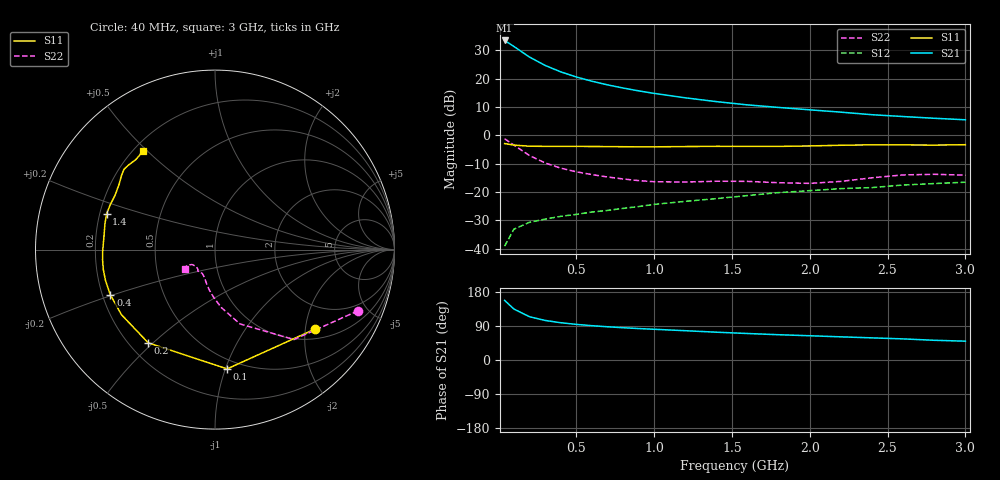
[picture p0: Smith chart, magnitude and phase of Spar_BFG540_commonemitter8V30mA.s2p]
! Filename:  BFG540J.S2P  Version:  3.0
! NXP part #: BFG540  Date: Feb 1992
! Bias condition: Vce=8V, Ic=30mA
! IN LINE PINNING: same data as with cross emitter pinning.
#  MHz  S  MA  R  50
! Freq  S11  S21  S12  S22  !GUM [dB]
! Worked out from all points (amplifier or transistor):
!   21 points, 40 MHz to 3 GHz, reference 50 ohm
!   highest |S21| = 33.4 dB at 40 MHz (marker M1)
!   |S21| within 3 dB of that: start of sweep to 123.3 MHz
!   unconditionally stable (mu >= 1): 825 MHz to end of sweep
!   at 300 MHz: K = 0.56, MSG = 27.1 dB, |S12| = -29.6 dB
!   at 1 GHz: K = 1.07, MAG = 18.0 dB, |S12| = -24.4 dB
!   at 3 GHz: K = 1.17, MAG = 8.5 dB, |S12| = -16.6 dB
!   lowest NFmin = 1.70 dB at 900 MHz
!   S11 on the Smith chart (normalised r, x): 40 MHz: 1.25, -2.25; 100 MHz: 0.42, -1.01; 200 MHz: 0.27, -0.48; 400 MHz: 0.23, -0.20; 1.4 GHz: 0.23, +0.15; 3 GHz: 0.24, +0.48
40  0.711 -38.6  46.95 157.3  0.011 71.0  0.866 -23.2
100  0.668 -84.2  36.73 134.4  0.022 54.4  0.667 -48.7
200  0.639 -125.6  23.9 114.2  0.029 44.8  0.437 -71.4
300  0.635 -145.2  17.04 104.4  0.033 43.9  0.324 -83.9
400  0.635 -156.7  13.12 98.4  0.037 45.6  0.262 -92.2
500  0.634 -164.3  10.66 94.0  0.04 48.0  0.226 -98.2
600  0.632 -170.0  8.973 90.6  0.044 50.8  0.202 -102.7
700  0.629 -174.9  7.74 87.7  0.047 53.0  0.183 -106.5
800  0.626 -179.1  6.807 85.2  0.051 54.8  0.169 -110.0
900  0.623 176.9  6.063 83.0  0.055 56.6  0.158 -113.9
1000  0.623 173.1  5.468 81.1  0.06 58.2  0.151 -118.0
1200  0.63 166.7  4.567 77.3  0.068 60.5  0.149 -125.2
1400  0.636 161.7  3.913 73.4  0.076 61.4  0.154 -128.4
1600  0.635 156.9  3.425 69.9  0.086 63.3  0.153 -129.1
1800  0.634 151.5  3.088 66.7  0.097 63.3  0.145 -131.1
2000  0.646 145.9  2.803 64.0  0.105 64.2  0.141 -138.6
2200  0.664 141.7  2.549 61.1  0.114 64.1  0.153 -147.1
2400  0.676 138.7  2.297 58.4  0.119 64.7  0.177 -150.5
2600  0.674 135.6  2.133 55.7  0.132 63.8  0.199 -148.7
2800  0.668 131.3  1.988 52.0  0.14 61.7  0.204 -146.2
3000  0.679 126.2  1.869 49.7  0.148 62.4  0.197 -147.6
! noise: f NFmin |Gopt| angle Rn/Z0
900  1.7  0.241  149  0.15
2000  2.4  0.479  -163  0.12
